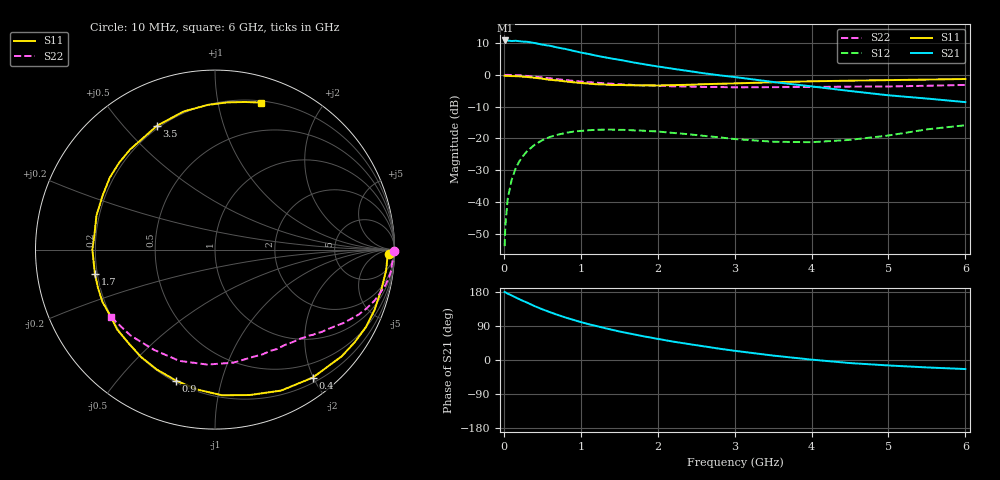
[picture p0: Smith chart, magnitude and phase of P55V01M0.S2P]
! SIEMENS Small Signal Semiconductors
! BFP183
! Si NPN RF Bipolar Junction Transistor in SOT143
! VCE = 5 V  IC = 1 mA
! Common Emitter S-Parameters:  March  1996
# GHz  S  MA  R  50
!  f  S11  S21  S12  S22
! GHz  MAG  ANG  MAG  ANG  MAG  ANG  MAG  ANG
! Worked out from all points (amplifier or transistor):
!   36 points, 10 MHz to 6 GHz, reference 50 ohm
!   highest |S21| = 10.8 dB at 20 MHz (marker M1)
!   |S21| within 3 dB of that: start of sweep to 856.7 MHz
!   unconditionally stable (mu >= 1): 2.504 GHz to end of sweep
!   at 250 MHz: K = 0.10, MSG = 18.0 dB, |S12| = -25.6 dB
!   at 1.4 GHz: K = 0.54, MSG = 11.2 dB, |S12| = -17.3 dB
!   at 6 GHz: K = 1.03, MAG = 2.5 dB, |S12| = -15.9 dB
!   S11 on the Smith chart (normalised r, x): 10 MHz: 41, -28; 400 MHz: 0.27, -1.99; 900 MHz: 0.21, -0.73; 1.7 GHz: 0.19, -0.10; 3.5 GHz: 0.19, +0.62; 6 GHz: 0.22, +1.34
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0.01  0.9673 -1.3  3.427 179.4  0.002 88.5  0.9999 -0.4
0.02  0.9615 -2.7  3.469 178.7  0.0042 87.2  0.9915 -0.9
0.05  0.9605 -6.8  3.458 175.2  0.0111 87.8  0.9958 -2.3
0.1  0.9534 -13.3  3.398 170.4  0.0218 81.1  0.9891 -4.7
0.15  0.9502 -20.6  3.43 165.5  0.0327 77.0  0.9874 -7.2
0.3  0.9229 -40.1  3.309 151.7  0.0622 65.6  0.958 -13.6
0.4  0.8974 -52.6  3.162 142.2  0.079 58.2  0.9338 -17.7
0.5  0.8675 -64.9  2.983 133.8  0.0933 51.4  0.9059 -21.2
0.6  0.8329 -76.6  2.858 126.2  0.1051 45.2  0.8786 -24.3
0.8  0.7859 -97.3  2.549 112.2  0.1212 34.3  0.8263 -29.6
0.9  0.7617 -106.5  2.387 106.1  0.1271 29.6  0.8012 -31.8
1.1  0.7263 -124.6  2.126 94.6  0.1338 21.6  0.7637 -35.8
1.4  0.6902 -147.9  1.802 80.1  0.1369 11.7  0.7226 -41.1
1.5  0.6914 -155.1  1.722 75.4  0.1358 9.2  0.7082 -42.6
1.7  0.6828 -168.5  1.552 67.3  0.1328 4.7  0.6883 -46.0
1.9  0.6833 179.8  1.413 59.5  0.1297 0.7  0.6761 -49.1
2.2  0.6872 163.9  1.243 48.6  0.1215 -3.3  0.6576 -54.2
2.8  0.7209 137.8  0.982 29.9  0.1035 -6.2  0.6412 -65.5
3.5  0.7618 115.1  0.77 11.7  0.0882 1.3  0.6384 -80.7
4.5  0.8073 92.8  0.555 -8.1  0.0944 20.0  0.651 -107.8
5.5  0.8396 78.4  0.422 -19.6  0.1381 27.3  0.6712 -134.6
6  0.8581 72.6  0.371 -23.9  0.1605 24.5  0.6918 -147.3
